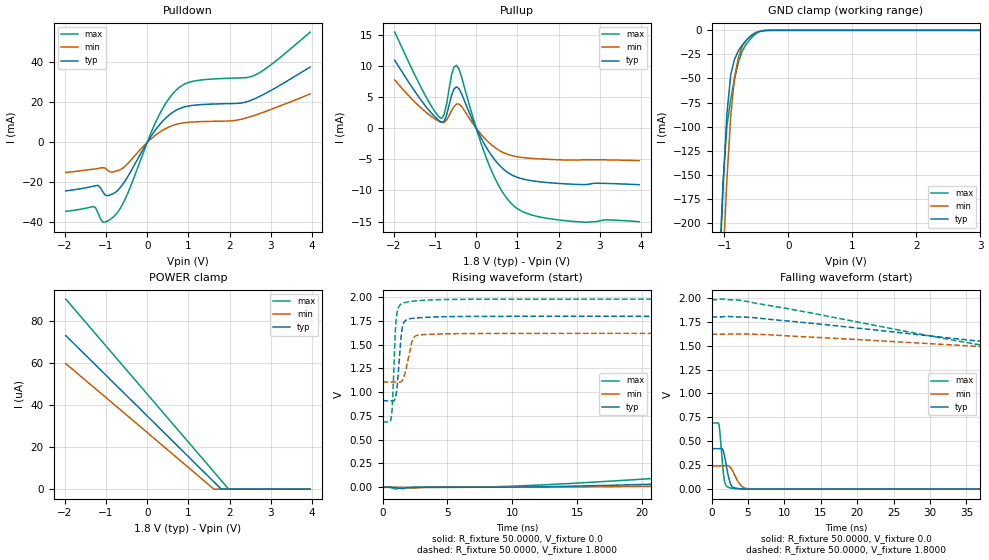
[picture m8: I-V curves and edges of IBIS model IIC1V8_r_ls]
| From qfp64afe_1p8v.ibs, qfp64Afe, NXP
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[Model] IIC1V8_r_ls
|   Model IIC1V8_r_ls
| This model was characterised for following simulation conditions:
| External (pad) voltage:
|   - Typ: 1.8V,   - Min: 1.62V,   - Max: 1.98V
| Library cells for typ/min/max conditions are connected as defined below:
|  IO - External Pad
|  A - Core Input
|  EN - Output Buffer Enable
|  BOOST - vdde
|  EGP - vdd
|  EHS - gnd
|  ENZI - vdd
|  EPD - vdd
|  EPUN - gnd
|  ZI - NC
|  ZIF - NC
|  gnd - gnd
|  gnde - gnde
|  vdd - vdd
|  vdde - vdde
| All other pins connected to ground
Model_type I/O
Polarity   Non-Inverting
Enable   Active-Low
Vinl =   0.5400V
Vinh =   1.2600V
Vmeas =  0.9000V
Cref =   0.0F
Rref =   1.0000k
Vref =   0.0V
C_comp   3.6136pF   3.4665pF   3.7543pF
|C_comp_pullup   0.9376pF   0.9156pF   0.9440pF
|C_comp_pulldown   2.3254pF   2.4783pF   2.1797pF
[Model Spec]
| variable   typ   min   max
Vinh   0.5400V   0.4860V   0.5940V
Vinl   1.2600V   1.1340V   1.3860V
Vmeas   0.9000V   0.8100V   0.9900V
[Temperature Range]   25.0000   0.1250k   -40.0000
[Voltage Range]   1.8000V   1.6200V   1.9800V
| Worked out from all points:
|   slope of the pulldown table from 0 to 0.27 V, typ, clamps not added: 33.4 ohm
|   slope of the pullup table from 0 to 0.27 V, typ, clamps not added: 80.7 ohm
|   GND clamp passes 1 mA (typ) near -0.44 V on its own axis
|   rising waveform, R_fixture 50.0000, V_fixture 0.0: 20-80 % time 70.1ns typ, 81.9ns min, 57ns max; typ from 0 V to 0.423 V
|   rising waveform, R_fixture 50.0000, V_fixture 1.8000: 20-80 % time 318ps typ, 487ps min, 235ps max; typ from 0.91 V to 1.8 V
|   falling waveform, R_fixture 50.0000, V_fixture 0.0: 20-80 % time 671ps typ, 1.04ns min, 474ps max; typ from 0.423 V to 0 V
|   falling waveform, R_fixture 50.0000, V_fixture 1.8000: 20-80 % time 66.9ns typ, 88.6ns min, 48.9ns max; typ from 1.8 V to 0.91 V
[Pulldown]
|Voltage   I(typ)   I(min)   I(max)
-1.98V    -24.22mA   -15.04mA   -34.42mA
-1.32V    -21.94mA   -13.4mA    -32.06mA
-1.2V     -21.45mA   -13.05mA   -35.06mA
-1.08V    -24.63mA   -12.6mA    -39.9mA
-900mV    -26.23mA   -14.78mA   -38.53mA
-720mV    -24.07mA   -14.13mA   -34.99mA
-540mV    -19.33mA   -11.9mA    -28.53mA
300mV     8.856mA    5.096mA    14.12mA
720mV     16.26mA    9.117mA    26.48mA
1.14V     18.6mA     10.26mA    30.69mA
2.58V     21.55mA    13.34mA    33.32mA
3.96V     37.7mA     24.26mA    55.17mA
[Pullup]
|Voltage   I(typ)   I(min)   I(max)
-1.98V    10.93mA    7.779mA    15.48mA
-1.32V    4.332mA    3.147mA    6.287mA
-900mV    1.21mA     1.087mA    1.795mA
-780mV    1.15mA     923.8uA    2.217mA
-600mV    5.282mA    2.828mA    8.607mA
-480mV    6.665mA    3.904mA    10.12mA
-420mV    6.371mA    3.888mA    9.538mA
360mV     -4.265mA   -2.608mA   -6.666mA
660mV     -6.57mA    -3.917mA   -10.5mA
960mV     -7.8mA     -4.537mA   -12.74mA
2.04V     -8.889mA   -5.075mA   -14.77mA
3.96V     -9.081mA   -5.209mA   -15.04mA
[GND_clamp]
|Voltage   I(typ)   I(min)   I(max)
-1.98V    -2.104A    -2.075A    -2.136A
-1.08V    -259.3mA   -333mA     -246.9mA
-1.02V    -161.8mA   -238.7mA   -157.1mA
-960mV    -86.75mA   -154.7mA   -99.47mA
-900mV    -45.96mA   -88.82mA   -71.06mA
-840mV    -29.91mA   -48mA      -50.26mA
-780mV    -21.16mA   -27.65mA   -32.99mA
-720mV    -15.17mA   -16.88mA   -21.27mA
-660mV    -10.57mA   -10.24mA   -14.57mA
-540mV    -3.796mA   -3.405mA   -5.301mA
-300mV    -21.69uA   -40.85uA   -23.15uA
3.96V     0A         0A         0A
[POWER_clamp]
|Voltage   I(typ)   I(min)   I(max)
-1.98V    73.06uA    59.72uA    90.42uA
1.62V     3.484uA    0A         8.225uA
1.8V      0A         0A         4.113uA
1.98V     0A         0A         0A
3.96V     0A         0A         0A
[Ramp]
| variable   typ   min   max
dV/dt_r  0.2537/70.0799n   0.1455/81.9024n   0.4146/57.0111n
dV/dt_f  0.5332/66.9050n   0.3065/88.6004n   0.7749/48.8984n
R_load = 50.0000
[Rising Waveform]
R_fixture= 50.0000
V_fixture= 0.0
V_fixture_min= 0.0
V_fixture_max= 0.0
|time   V(typ)   V(min)   V(max)
0s        583.8pV    50.78nV    39.11pV
1.016ns   -3.394mV   194.4uV    -19.97mV
1.641ns   -11.01mV   -2.853mV   -1.751mV
12.85ns   6.697mV    1.515mV    28.34mV
46.96ns   150.1mV    67.36mV    312.8mV
85.54ns   288mV      145mV      565.7mV
105.4ns   345mV      174.9mV    633.5mV
136.3ns   394.1mV    209.7mV    673.5mV
254.6ns   422mV      241.2mV    690.6mV
1us       422.8mV    242.6mV    690.9mV
[Rising Waveform]
R_fixture= 50.0000
V_fixture= 1.8000
V_fixture_min= 1.6200
V_fixture_max= 1.9800
|time   V(typ)   V(min)   V(max)
0s        910.3mV    1.108V     687.5mV
676.9ps   909mV      1.108V     736.7mV
774.7ps   906.6mV    1.108V     909.4mV
1.009ns   951.8mV    1.107V     1.697V
1.276ns   1.316V     1.104V     1.905V
1.482ns   1.642V     1.117V     1.931V
1.774ns   1.755V     1.22V      1.945V
2.482ns   1.779V     1.585V     1.959V
5.847ns   1.796V     1.615V     1.976V
1us       1.799V     1.619V     1.979V
[Falling Waveform]
R_fixture= 50.0000
V_fixture= 0.0
V_fixture_min= 0.0
V_fixture_max= 0.0
|time   V(typ)   V(min)   V(max)
0s        422.9mV    242.6mV    691mV
997.6ps   422.8mV    242.6mV    678mV
1.154ns   424.1mV    242.6mV    586mV
1.627ns   396.7mV    242.7mV    161.6mV
1.947ns   277.7mV    244.3mV    43.48mV
2.362ns   116.8mV    241.2mV    17.53mV
2.776ns   30.54mV    207.8mV    9.765mV
4.029ns   4.312mV    38.02mV    3.075mV
5.124ns   1.721mV    4.651mV    1.74mV
1us       18.99nV    83.33nV    10.91nV
[Falling Waveform]
R_fixture= 50.0000
V_fixture= 1.8000
V_fixture_min= 1.6200
V_fixture_max= 1.9800
|time   V(typ)   V(min)   V(max)
0s        1.799V     1.619V     1.979V
4.163ns   1.799V     1.622V     1.972V
58.09ns   1.392V     1.406V     1.242V
67.68ns   1.33V      1.372V     1.004V
75.64ns   1.277V     1.346V     873.8mV
91.82ns   1.112V     1.297V     759.5mV
112.7ns   987.5mV    1.233V     712mV
146.3ns   930mV      1.146V     692.6mV
204.6ns   913mV      1.113V     688.1mV
1us       910.4mV    1.108V     687.5mV
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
